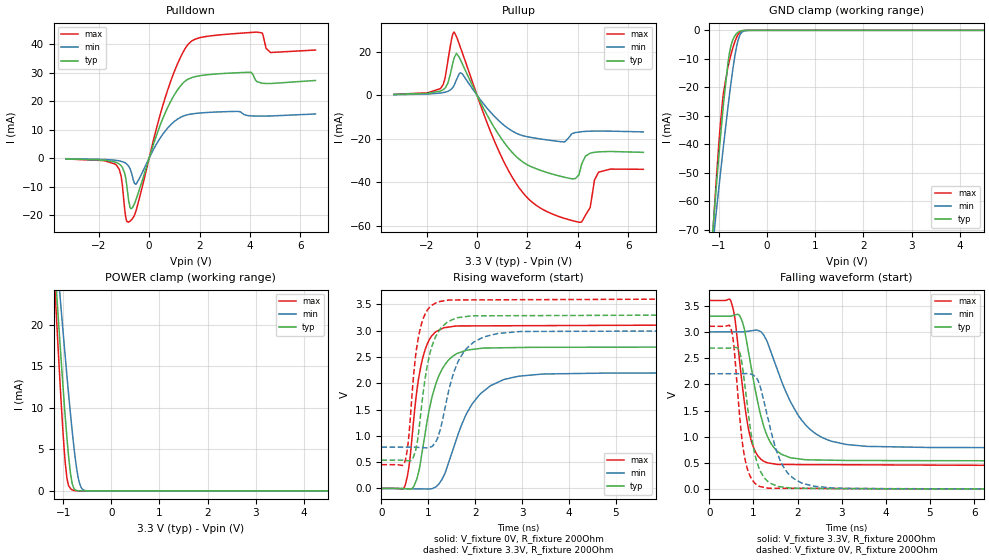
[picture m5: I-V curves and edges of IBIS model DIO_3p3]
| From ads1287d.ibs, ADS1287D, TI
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|   Model
[Model]   DIO_3p3
Model_type   I/O
Polarity   Non-Inverting
Enable   Active-Low
Vinl = 0.99
Vinh = 2.31
Vmeas = 1.65
Vref = 0
Cref = 1pF
Rref = 100000
|   typ   min   max
C_comp   3.504pF   3.036pF   3.899p
[Voltage Range]   3.3   3   3.6
[Temperature Range]   27   125   -40
[Pullup Reference]   3.3   3   3.6
[Pulldown Reference]   -0   0   0
[Power Clamp Reference]   3.3   3   3.6
[GND Clamp Reference]   0   0   0
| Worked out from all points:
|   slope of the pulldown table from 0 to 0.495 V, typ, clamps not added: 38.4 ohm
|   slope of the pullup table from 0 to 0.495 V, typ, clamps not added: 44.6 ohm
|   GND clamp passes 1 mA (typ) near -0.63 V on its own axis
|   POWER clamp passes 1 mA (typ) near -0.82 V on its own axis
|   falling waveform, V_fixture 3.3V, R_fixture 200Ohm: 20-80 % time 418ps typ, 758ps min, 285ps max; typ from 3.3 V to 0.537 V
|   rising waveform, V_fixture 0V, R_fixture 200Ohm: 20-80 % time 392ps typ, 660ps min, 267ps max; typ from 0 V to 2.69 V
|   rising waveform, V_fixture 3.3V, R_fixture 200Ohm: 20-80 % time 299ps typ, 446ps min, 218ps max; typ from 0.537 V to 3.3 V
|   falling waveform, V_fixture 0V, R_fixture 200Ohm: 20-80 % time 294ps typ, 456ps min, 215ps max; typ from 2.69 V to 0 V
[Pulldown]
|   Voltage   I(typ)   I(min)   I(max)
-3.3V     -275.6uA   -195.7uA   -299.3uA
-1.3V     -1.554mA   -799.9uA   -2.487mA
-1.112V   -2.678mA   -1.126mA   -6.45mA
-973.5mV  -5.253mA   -1.591mA   -17.71mA
-815.1mV  -14.84mA   -2.807mA   -22.53mA
-518.1mV  -14.5mA    -9.101mA   -18.41mA
709.5mV   17.33mA    10.32mA    23.26mA
1.68V     28.27mA    15.51mA    41.13mA
4.036V    30.16mA    14.85mA    44.18mA
4.274V    26.91mA    14.79mA    44.31mA
4.818V    26.22mA    14.81mA    37.13mA
6.6V      27.31mA    15.52mA    38.01mA
[GND Clamp]
|   Voltage   I(typ)   I(min)   I(max)
-3.3V     -599.4mA   -485.7mA   -710.1mA
-1.191V   -84.36mA   -85.93mA   -88.3mA
-1.092V   -62.69mA   -69.53mA   -61.73mA
-1.063V   -56.38mA   -64.74mA   -54.12mA
-983.4mV  -40.18mA   -52.28mA   -35.43mA
-904.2mV  -25.38mA   -40.2mA    -21.67mA
-815.1mV  -11.64mA   -27.19mA   -13mA
-755.7mV  -5.782mA   -19.09mA   -8.839mA
-656.7mV  -1.607mA   -7.686mA   -3.378mA
-567.6mV  -321.1uA   -1.751mA   -709.4uA
-280.5mV  -304.9nA   -1.84uA    -326.4nA
6.6V      0A         0A         0A
[Pullup]
|   Voltage   I(typ)   I(min)   I(max)
-3.3V     368uA      267.7uA    426.8uA
-1.439V   2mA        1.043mA    3.272mA
-1.162V   5.493mA    1.817mA    15.57mA
-914.1mV  17.01mA    4.509mA    29.11mA
-617.1mV  15.27mA    10.16mA    20.63mA
986.7mV   -20.32mA   -13mA      -28.77mA
2.373V    -33.95mA   -19.86mA   -50.87mA
3.769V    -38.49mA   -17.67mA   -57.69mA
4.125V    -32.95mA   -16.81mA   -58.46mA
4.481V    -26.73mA   -16.54mA   -51.86mA
4.818V    -26.06mA   -16.49mA   -35.49mA
6.6V      -26.28mA   -16.86mA   -34.09mA
[POWER Clamp]
|   Voltage   I(typ)   I(min)   I(max)
-3.3V     229.1mA    189.8mA    280.5mA
-1.181V   27.94mA    31.67mA    25.63mA
-1.122V   22.68mA    27.48mA    19.07mA
-1.063V   17.55mA    23.35mA    12.8mA
-1.003V   12.6mA     19.29mA    7.07mA
-953.7mV  8.726mA    15.98mA    3.213mA
-904.2mV  5.227mA    12.77mA    1.002mA
-844.8mV  1.982mA    9.099mA    254.1uA
-805.2mV  748.3uA    6.819mA    111.6uA
-676.5mV  17.54uA    1.311mA    8.746uA
-528mV    3.87uA     32.31uA    5.059uA
6.6V      0A         0A         0A
[Ramp]
R_load = 200
|   typ   min   max
dV/dt_r   1.61405/3.89639e-10   1.32016/6.54733e-10   1.86425/2.67051e-10
dV/dt_f   1.65766/4.16021e-10   1.32901/7.56248e-10   1.88889/2.83919e-10
[Falling Waveform]
V_fixture = 3.3V
V_fixture_min = 3V
V_fixture_max = 3.6V
R_fixture = 200Ohm
C_fixture = 0F
|   Time   V(typ)   V(min)   V(max)
0s        3.3V       3V         3.6V
490.4ps   3.301V     3V         3.584V
696.2ps   3.296V     3V         2.361V
842.9ps   2.824V     3.009V     1.359V
996.9ps   2.094V     3.027V     803.1mV
1.25ns    1.152V     2.911V     525.3mV
1.536ns   727mV      2.29V      472.6mV
2.33ns    558.1mV    1.107V     468.1mV
3.587ns   545.9mV    815.8mV    464mV
50ns      537.1mV    784.9mV    451.7mV
[Rising Waveform]
V_fixture = 0V
V_fixture_min = 0V
V_fixture_max = 0V
R_fixture = 200Ohm
C_fixture = 0F
|   Time   V(typ)   V(min)   V(max)
0s        -639.3nV   98.36nV    -30.06nV
490.4ps   -2.573mV   -5.156mV   26.91mV
598.6ps   -12mV      -6.294mV   488.6mV
696.2ps   48.91mV    -7.32mV    1.378V
976.4ps   1.286V     -10.27mV   2.744V
1.222ns   2.133V     81.03mV    3.005V
1.579ns   2.546V     878mV      3.086V
2.33ns    2.671V     1.954V     3.091V
3.501ns   2.683V     2.176V     3.095V
50ns      2.69V      2.2V       3.107V
[Rising Waveform]
V_fixture = 3.3V
V_fixture_min = 3V
V_fixture_max = 3.6V
R_fixture = 200Ohm
C_fixture = 0F
|   Time   V(typ)   V(min)   V(max)
0s        537.1mV    784.9mV    451.7mV
490.4ps   533.1mV    785.1mV    484.5mV
577ps     525mV      785.1mV    924.7mV
666.4ps   562.3mV    785.2mV    1.936V
900.7ps   1.89V      774.4mV    3.251V
1.188ns   2.933V     935.6mV    3.539V
1.436ns   3.178V     1.854V     3.581V
1.972ns   3.281V     2.783V     3.584V
3.015ns   3.285V     2.984V     3.588V
50ns      3.3V       3V         3.6V
[Falling Waveform]
|Gnd
V_fixture = 0V
V_fixture_min = 0V
V_fixture_max = 0V
R_fixture = 200Ohm
C_fixture = 0F
|   Time   V(typ)   V(min)   V(max)
0s        2.69V      2.2V       3.107V
481.6ps   2.692V     2.202V     3.091V
654ps     2.677V     2.203V     1.722V
758.9ps   2.283V     2.204V     820.4mV
881.9ps   1.459V     2.204V     335.3mV
1.055ns   584.3mV    2.135V     96.41mV
1.332ns   143.4mV    1.334V     18.72mV
1.788ns   25.81mV    297.8mV    16.16mV
2.928ns   9.111mV    18.08mV    13.06mV
50ns      34.82nV    156nV      -25.33nV
